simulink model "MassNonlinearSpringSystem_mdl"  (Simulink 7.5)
settings: Solver=ode45  StartTime=0.0  StopTime=10.0  MaxStep=1e-2  RelTol=1e-3
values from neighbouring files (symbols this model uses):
  b = 0.01    [Exercises04a.m]    (also in Exercises04b.m = 0.75)
  dx0 = xe(1)    [Exercises04b.m]
  k0 = 0.5    [Exercises04b.m]
  k1 = 0.25    [Exercises04b.m]
  m = 1    [Exercises04b.m]
  x0 = [70; 70]    [Exercises04a.m]    (also in Exercises04b.m = xe(2))

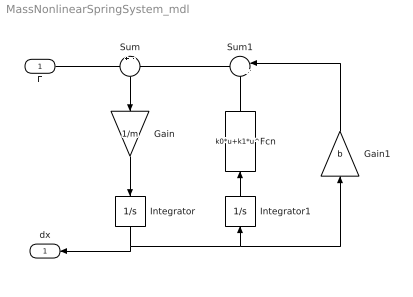
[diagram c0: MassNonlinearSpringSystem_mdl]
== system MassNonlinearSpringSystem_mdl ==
  F : Inport  OutDataType=sfix(16)  OutScaling=2^0
  Fcn : Fcn  Expr=k0*u+k1*u^3
  Gain : Gain  Gain=1/m  ParameterDataType=sfix(16)  ParameterScaling=2^0  OutDataType=sfix(16)  OutScaling=2^0
  Gain1 : Gain  Gain=b  ParameterDataType=sfix(16)  ParameterScaling=2^0  OutDataType=sfix(16)  OutScaling=2^0
  Integrator : Integrator  InitialCondition=dx0
  Integrator1 : Integrator  InitialCondition=x0
  Sum : Sum  Inputs=+-  OutDataType=sfix(16)  OutScaling=2^0
  Sum1 : Sum  Inputs=|++  OutDataType=sfix(16)  OutScaling=2^0
  dx : Outport  OutDataType=sfix(16)  OutScaling=2^0
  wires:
  Gain/1 -> Integrator/1
  Sum/1 -> Gain/1
  Integrator/1 -> dx/1, Integrator1/1, Gain1/1
  Sum1/1 -> Sum/2
  Fcn/1 -> Sum1/2
  Gain1/1 -> Sum1/1
  Integrator1/1 -> Fcn/1
  F/1 -> Sum/1
